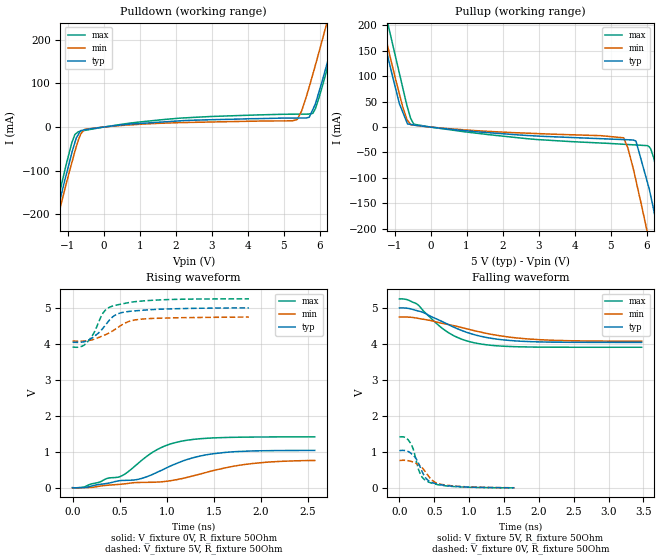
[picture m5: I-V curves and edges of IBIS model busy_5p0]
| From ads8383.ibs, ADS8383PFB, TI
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|   busy_5p0 Model
[Model]   busy_5p0
Model_type   Output
Polarity   Non-Inverting
Vmeas = 2.5
Vref = 2.5
Cref = 20pF
Rref = 50
|   typ   min   max
|   (nom PVT)   (fast PVT)   (slow PVT)
|C_comp from frequency sweep method (F=500KHz)
|C_comp   1.966e-12   1.871e-12   2.054e-12
|ON state : BUFFER OUTPUT TURNED HIGH
|C_comp   1.966e-12   1.871e-12   2.054e-12
|OFF state: BUFFER OUTPUT TURNED LOW
|C_comp   2.070e-12   1.997e-12   2.132e-12
|C_comp from LC tank measurement(L=1nH)
|Resonant Frequency(Hz)   6.790e+09   6.960e+09   6.560e+09
C_comp   5.500e-13   5.234e-13   5.892e-13
|ON state : BUFFER OUTPUT TURNED HIGH
|Resonant Frequency(Hz)   6.790e+09   6.960e+09   6.560e+09
|C_comp   5.500e-13   5.234e-13   5.892e-13
|OFF state: BUFFER OUTPUT TURNED LOW
|Resonant Frequency(Hz)   6.840e+09   7.030e+09   6.600e+09
|C_comp   5.420e-13   5.131e-13   5.821e-13
| Where nom  PVT is Nominal Process, 5V, 35C
|   Fast PVT is Strong Process,  5.25V, -30C
|   Slow PVT is Weak Process,   4.75V, 95C
[Voltage Range]   5   4.75   5.25
|Ambient Temperature   25   85   -40
|Junction Temperature
[Temperature Range]   35   95   -40
[Pullup Reference]   5   4.75   5.25
[Pulldown Reference]   0   0   0
[Power Clamp Reference]   5   4.75   5.25
[GND Clamp Reference]   0   0   0
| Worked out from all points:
|   slope of the pulldown table from 0 to 0.75 V, typ, clamps not added: 109 ohm
|   slope of the pullup table from 0 to 0.75 V, typ, clamps not added: 131 ohm
|   falling waveform, V_fixture 5V, R_fixture 50Ohm: 20-80 % time 710ps typ, 976ps min, 522ps max; typ from 5 V to 4.04 V
|   rising waveform, V_fixture 0V, R_fixture 50Ohm: 20-80 % time 673ps typ, 879ps min, 502ps max; typ from 0 V to 1.04 V
|   rising waveform, V_fixture 5V, R_fixture 50Ohm: 20-80 % time 216ps typ, 277ps min, 172ps max; typ from 4.04 V to 5 V
|   falling waveform, V_fixture 0V, R_fixture 50Ohm: 20-80 % time 179ps typ, 214ps min, 145ps max; typ from 1.04 V to 0.006 V
[Pulldown]
|   Voltage   I(typ)   I(min)   I(max)
-5V       -1.509A    -1.491A    -1.553A
-2.53V    -628.3mA   -634.7mA   -629.9mA
-1.31V    -199.8mA   -218.9mA   -180.5mA
-882mV    -58.79mA   -81.05mA   -35.37mA
-760mV    -24.93mA   -44.82mA   -14.38mA
-527.2mV  -6.318mA   -5.311mA   -7.682mA
5.372V    20.67mA    17.2mA     29.55mA
5.812V    40.63mA    121.5mA    31.86mA
6.075V    106.7mA    200.3mA    93.61mA
6.3V      174mA      269.7mA    161.3mA
6.525V    243mA      339mA      231mA
10V       1.346A     1.44A      1.339A
[Pullup]
|   Voltage   I(typ)   I(min)   I(max)
-5V       1.346A     1.361A     1.419A
-1.31V    176.2mA    195mA      241.2mA
-1.088V   109.2mA    128.1mA    173.6mA
-865mV    45.96mA    65.21mA    105.8mA
-541.5mV  5.051mA    4.491mA    15.69mA
5.358V    -24.6mA    -21.08mA   -33.78mA
5.705V    -27.43mA   -104.7mA   -35.21mA
6.009V    -104.9mA   -202.5mA   -36.47mA
6.116V    -135.5mA   -238.7mA   -42.91mA
6.3V      -197.2mA   -300.5mA   -91.57mA
6.57V     -290.3mA   -391.4mA   -185.2mA
10V       -1.509A    -1.577A    -1.459A
[Ramp]
R_load = 50
|   typ   min   max
dV/dt_r   0.622968/6.714e-10   0.45871/8.74986e-10   0.8491/5.02317e-10
dV/dt_f   0.573415/7.10183e-10   0.403668/9.77588e-10   0.804283/5.21735e-10
[Falling Waveform]
V_fixture = 5V
V_fixture_min = 4.75V
V_fixture_max = 5.25V
R_fixture = 50Ohm
|   Time   V(typ)   V(min)   V(max)
0s        5V         4.75V      5.25V
100ps     4.995V     4.749V     5.238V
250ps     4.926V     4.719V     5.112V
550ps     4.68V      4.6V       4.539V
750ps     4.495V     4.522V     4.262V
900ps     4.37V      4.454V     4.129V
1.1ns     4.245V     4.359V     4.023V
1.45ns    4.123V     4.226V     3.943V
1.925ns   4.062V     4.13V      3.915V
3.475ns   4.044V     4.078V     3.909V
[Rising Waveform]
V_fixture = 0V
V_fixture_min = 0V
V_fixture_max = 0V
R_fixture = 50Ohm
|   Time   V(typ)   V(min)   V(max)
0s        3.64nV     5.719nV    3.437nV
125ps     5.442mV    1.737mV    20.29mV
375ps     122.3mV    69.11mV    265.3mV
500ps     195mV      93.45mV    303.2mV
700ps     234.8mV    145.1mV    683.1mV
875ps     398.6mV    153.4mV    1.023V
1.15ns    720.7mV    246.4mV    1.289V
1.65ns    987.2mV    565.5mV    1.397V
2.075ns   1.029V     711.1mV    1.411V
2.575ns   1.036V     757mV      1.414V
[Rising Waveform]
V_fixture = 5V
V_fixture_min = 4.75V
V_fixture_max = 5.25V
R_fixture = 50Ohm
|   Time   V(typ)   V(min)   V(max)
0s        4.044V     4.077V     3.909V
100ps     4.047V     4.075V     3.931V
150ps     4.078V     4.084V     4.025V
225ps     4.196V     4.124V     4.289V
325ps     4.438V     4.226V     4.861V
375ps     4.607V     4.283V     4.993V
425ps     4.747V     4.356V     5.049V
575ps     4.892V     4.597V     5.135V
700ps     4.923V     4.676V     5.181V
1.875ns   4.998V     4.744V     5.249V
[Falling Waveform]
V_fixture = 0V
V_fixture_min = 0V
V_fixture_max = 0V
R_fixture = 50Ohm
|   Time   V(typ)   V(min)   V(max)
0s        1.038V     764.5mV    1.415V
75ps      1.041V     769.6mV    1.409V
150ps     986.1mV    748.7mV    1.273V
200ps     907.6mV    717.7mV    1.071V
300ps     573.4mV    611.8mV    386.2mV
375ps     283.2mV    442mV      211.1mV
425ps     193.6mV    309.2mV    160.3mV
525ps     118.7mV    146.1mV    102.6mV
700ps     62.23mV    72.59mV    53.57mV
1.65ns    6.022mV    7.344mV    4.57mV
